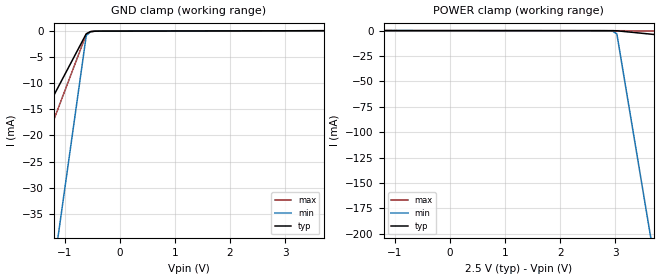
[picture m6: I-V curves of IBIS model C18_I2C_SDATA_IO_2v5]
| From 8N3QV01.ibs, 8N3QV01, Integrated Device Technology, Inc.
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[Model] C18_I2C_SDATA_IO_2v5
Model_type   Input
Polarity   Non-Inverting
Vinl = 0.7V
Vinh = 1.7V
|   typ   min   max
C_comp   2pF   1.5pF   2.5pF
|   typ   min   max
[Voltage range]   2.5V   2.375V   2.625V
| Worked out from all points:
|   GND clamp passes 1 mA (typ) near -0.63 V on its own axis
[GND_clamp]
|Voltage   I (typ)   I (min)   I (max)
-2.5V     -38.44mA   -143.2mA   -53.29mA
-2.424V   -36.93mA   -137.5mA   -51.19mA
-1.97V    -27.84mA   -103.3mA   -38.56mA
-1.894V   -26.32mA   -97.64mA   -36.45mA
-1.136V   -11.17mA   -40.73mA   -15.4mA
-1.061V   -9.653mA   -35.04mA   -13.29mA
-606.1mV  -561.9uA   -894.9uA   -660.6uA
-530.3mV  -155.5uA   -183.2uA   -155.3uA
-303mV    -56.19uA   -50.54uA   -62.19uA
5V        49.97uA    49.09uA    50.42uA
[Power_clamp]
|Voltage   I (typ)   I (min)   I (max)
-2.5V     49.97uA    46.75uA    53.08uA
2.955V    -73.26uA   -484.1uA   -62.81uA
3.03V     -155.5uA   -3.162mA   -65.88uA
3.561V    -3.001mA   -176mA     -211.6uA
3.636V    -3.407mA   -200.7mA   -232.4uA
5V        -10.72mA   -645.2mA   -607uA
